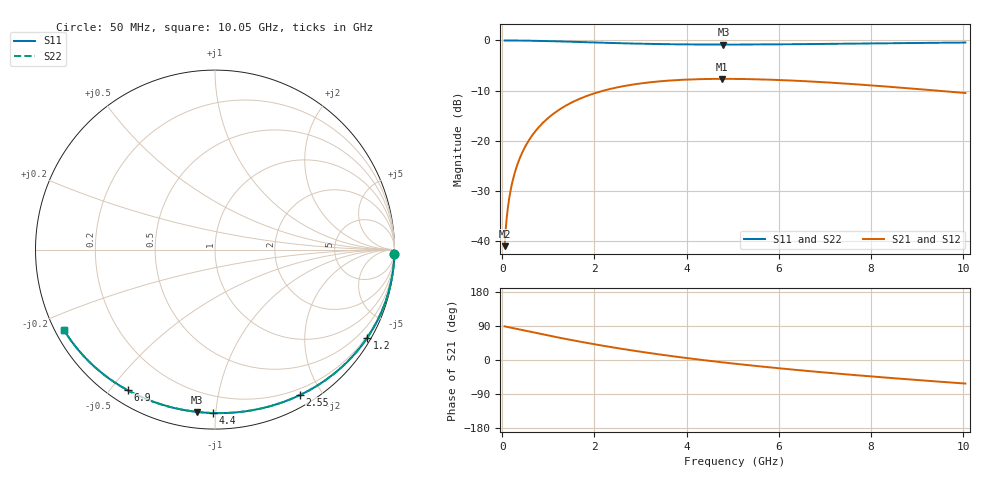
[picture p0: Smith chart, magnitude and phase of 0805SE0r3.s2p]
! AVX Thin Film Operation		Date: August 2001
! Description: Accu-P® Series, Thin Film, SMD, RF Capacitor
! Part Number: 08051J0R3ABT
! 50 MHz  -  10.05 GHz
! Serial Measurements
# mhz S db R 50
!	S11		S21		S12		S22
!	dB	Phase	dB	Phase	dB	Phase	dB	Phase
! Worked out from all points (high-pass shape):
!   401 points, 50 MHz to 10.05 GHz, reference 50 ohm
!   highest |S21| = -7.66 dB at 4.775 GHz (marker M1); lowest = -41.0 dB at 50 MHz (marker M2)
!   |S21| within 3 dB of the highest: 1.962 GHz to end of sweep
!   lowest |S11| = -0.8 dB at 4.8 GHz (marker M3), VSWR 21.20, Z = 4.23 - j44.5 ohm
!   |S11| at or under -10 dB: nowhere
!   |S22| runs from -0.8 to 0.0 dB; largest |S21 - S12| = 0
!   S11 on the Smith chart (normalised r, x): 50 MHz: 0, -88; 1.2 GHz: 0.15, -3.69; 2.55 GHz: 0.13, -1.74; 4.4 GHz: 0.09, -0.98; 6.9 GHz: 0.05, -0.55; 10.05 GHz: 0.03, -0.25
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50  -0.00 -1.3  -41.02 88.7  -41.02 88.7  -0.00 -1.3
75  -0.00 -1.9  -37.49 88.1  -37.49 88.1  -0.00 -1.9
150  -0.00 -3.9  -31.48 86.1  -31.48 86.1  -0.00 -3.9
200  -0.01 -5.2  -28.99 84.8  -28.99 84.8  -0.01 -5.2
300  -0.01 -7.8  -25.49 82.2  -25.49 82.2  -0.01 -7.8
400  -0.02 -10.3  -23.02 79.7  -23.02 79.7  -0.02 -10.3
550  -0.04 -14.2  -20.32 75.8  -20.32 75.8  -0.04 -14.2
725  -0.07 -18.6  -18.01 71.4  -18.01 71.4  -0.07 -18.6
950  -0.12 -24.2  -15.83 65.8  -15.83 65.8  -0.12 -24.2
1200  -0.18 -30.3  -14.02 59.7  -14.02 59.7  -0.18 -30.3
1725  -0.32 -42.4  -11.46 47.6  -11.46 47.6  -0.32 -42.4
2125  -0.44 -51.1  -10.19 38.9  -10.19 38.9  -0.44 -51.1
2550  -0.55 -59.7  -9.25 30.3  -9.25 30.3  -0.55 -59.7
3400  -0.72 -75.1  -8.16 14.9  -8.16 14.9  -0.72 -75.1
4400  -0.81 -90.8  -7.69 -0.8  -7.69 -0.8  -0.81 -90.8
4775  -0.82 -96.1  -7.66 -6.1  -7.66 -6.1  -0.82 -96.1
4800  -0.82 -96.4  -7.66 -6.5  -7.66 -6.5  -0.82 -96.5
5050  -0.82 -99.8  -7.67 -9.9  -7.67 -9.9  -0.82 -99.8
6725  -0.72 -120.0  -8.20 -30.0  -8.20 -30.0  -0.72 -120.0
6900  -0.70 -121.9  -8.29 -32.0  -8.29 -32.0  -0.70 -121.9
8400  -0.56 -137.1  -9.23 -47.2  -9.23 -47.2  -0.56 -137.1
10050  -0.42 -152.0  -10.48 -62.2  -10.48 -62.2  -0.42 -152.1
